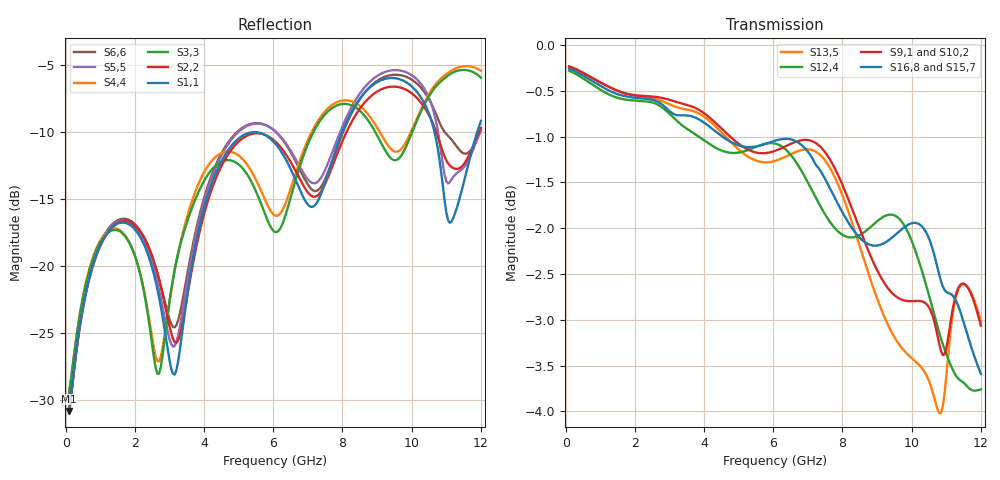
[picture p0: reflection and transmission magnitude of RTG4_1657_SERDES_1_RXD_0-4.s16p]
! RTG4 1657 S-parameter file
! Microsemi Corporation (c) 2019
!Initial ver: Jul 30, 2019
! Port::PIN_NAME::NET_NAME::S-parameter ports::PORT SIDE
! Port1:--:SERDES_1_RXD0_N_DIE::1::DIE
! Port2:--:SERDES_1_RXD0_P_DIE::2::DIE
! Port3:AW10:SERDES_1_RXD0_N_BGA::3::BGA
! Port4:AV10:SERDES_1_RXD0_P_BGA::4::BGA
! Port5:--:SERDES_1_RXD1_N_DIE::5::DIE
! Port6:--:SERDES_1_RXD1_P_DIE::6::DIE
! Port7:BA11:SERDES_1_RXD1_N_BGA::7::BGA
! Port8:AY11:SERDES_1_RXD1_P_BGA::8::BGA
! Port9:--:SERDES_1_RXD2_N_DIE::9::DIE
! Port10:--:SERDES_1_RXD2_P_DIE::10::DIE
! Port11:AW12:SERDES_1_RXD2_N_BGA::11::BGA
! Port12:AV12:SERDES_1_RXD2_P_BGA::12::BGA
! Port13:--:SERDES_1_RXD3_N_DIE::13::DIE
! Port14:--:SERDES_1_RXD3_P_DIE::14::DIE
! Port15:BA13:SERDES_1_RXD3_N_BGA::15::BGA
! Port16:AY13:SERDES_1_RXD3_P_BGA::16::BGA
!TouchstoneFormatFlag = 1
! GNDNET
! NETSLIST
! User Comments:
! Touchstone file exported from HFSS 2018.2.0
!  File:  C:/Users/LSI_SIM_01/Desktop/Microsemi_190710/YBD197_150320_NETCHANGE_SERDES_1_RXD.aedt
!  Generated:  1:05:42 ??  7 12, 2019
!  Design:  HFSSModel1
!  Project:  YBD197_150320_NETCHANGE_SERDES_1_RXD
!  Setup:  Setup1
!  Solution:  Sweep
! Terminal data exported
! Port[1] = SERDES_1_RXD0_N_DIE
! Port[2] = SERDES_1_RXD0_P_DIE
! Port[3] = SERDES_1_RXD1_N_DIE
! Port[4] = SERDES_1_RXD1_P_DIE
! Port[5] = SERDES_1_RXD2_N_DIE
! Port[6] = SERDES_1_RXD2_P_DIE
! Port[7] = SERDES_1_RXD3_N_DIE
! Port[8] = SERDES_1_RXD3_P_DIE
! Port[9] = SERDES_1_RXD0_N_BGA
! Port[10] = SERDES_1_RXD0_P_BGA
! Port[11] = SERDES_1_RXD1_N_BGA
! Port[12] = SERDES_1_RXD1_P_BGA
! Port[13] = SERDES_1_RXD2_N_BGA
! Port[14] = SERDES_1_RXD2_P_BGA
! Port[15] = SERDES_1_RXD3_N_BGA
! Port[16] = SERDES_1_RXD3_P_BGA
# GHZ S DB R 50.000000
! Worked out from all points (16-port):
!   239 points, 100 MHz to 12 GHz, reference 50 ohm
!   strongest paths, dB at 100 MHz, 3.05 GHz, 6.05 GHz, 9.05 GHz, 12 GHz:
!     S16,8: -0.3, -0.7, -1.0, -2.2, -3.6
!     S9,1: -0.2, -0.6, -1.2, -2.5, -3.1
!     S15,7: -0.3, -0.8, -1.1, -2.4, -3.8
!     S12,4: -0.3, -0.8, -1.1, -1.9, -3.8
!     S13,5: -0.2, -0.7, -1.3, -2.8, -3.0
!     S10,2: -0.2, -0.6, -1.2, -2.6, -3.1
!   lowest |S11| = -30.8 dB at 100 MHz (marker M1), VSWR 1.06, Z = 52.5 - j1.56 ohm
!   |S11| at or under -10 dB: start of sweep to 7.997 GHz; 10.66 GHz to 11.89 GHz (1.235 GHz wide, 11 % of centre)
